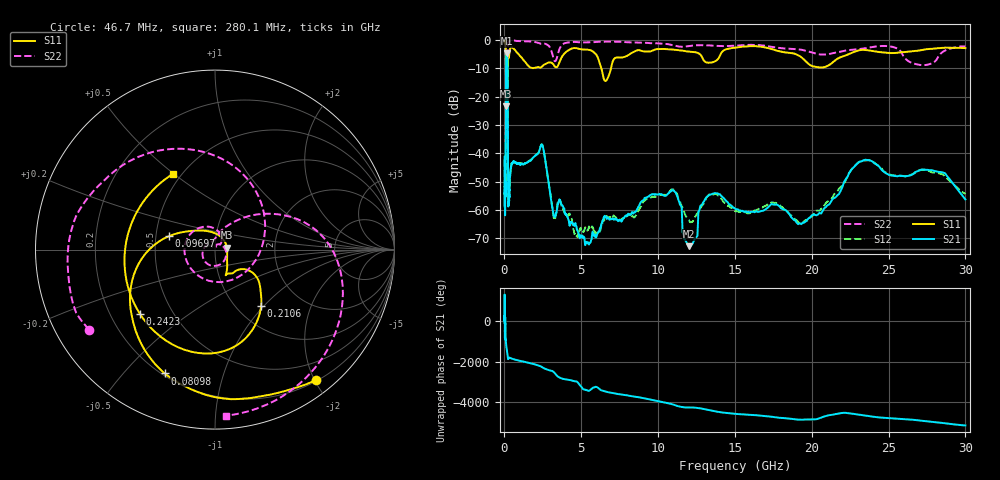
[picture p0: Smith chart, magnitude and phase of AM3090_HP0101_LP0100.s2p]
! Date/Time: Thu, Feb 28, 2019 1:58 PM
! Network Analyzer: Agilent Technologies E8364B Rev: A.07.50.67
! Sweep from 0.010 to 30.000 GHz, 1601 Points, Sweep Type: LOG
! Power Supply: 5.023 V, 0.002 A
# Hz S DB R 50
!freq MagS11 AngS11 MagS21 AngS21 MagS12 AngS12 MagS22 AngS22
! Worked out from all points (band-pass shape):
!   1601 points, 10 MHz to 30 GHz, reference 50 ohm
!   highest |S21| = -4.62 dB at 146.9 MHz (marker M1); lowest = -72.8 dB at 12.01 GHz (marker M2)
!   |S21| within 3 dB of the highest: 106.9 MHz to 197.1 MHz (90.2 MHz wide, 59.3 % of centre)
!   lowest |S11| = -23.4 dB at 105.1 MHz (marker M3), VSWR 1.14, Z = 57.1 + j1.3 ohm
!   |S11| at or under -10 dB: 96.08 MHz to 200.4 MHz (104.3 MHz wide, 70.4 % of centre); 6.307 GHz to 6.931 GHz (624.1 MHz wide, 9.43 % of centre)
!   |S22| runs from -34.9 to -0.1 dB; largest |S21 - S12| = 0.012
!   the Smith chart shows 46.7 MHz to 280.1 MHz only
!   S11 on the Smith chart (normalised r, x): 46.7 MHz: 0.22, -2.02; 80.98 MHz: 0.21, -0.65; 96.97 MHz: 0.58, +0.09; 210.6 MHz: 1.28, -0.96; 242.3 MHz: 0.33, -0.33; 280.1 MHz: 0.45, +0.49
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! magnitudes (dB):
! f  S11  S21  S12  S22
! 10 MHz  -0.3  -41.2  -42.2  -0.6
! 38.04 MHz  -0.5  -59.4  -60.7  -1.3
! 46.7 MHz  -0.8  -51.0  -50.0  -1.6
! 80.98 MHz  -2.6  -49.3  -49.0  -5.2
! 96.97 MHz  -11.4  -15.9  -15.9  -15.0
! 105.1 MHz  -23.4  -8.3  -8.3  -15.9
! 130.3 MHz  -16.3  -4.9  -4.9  -34.8
! 144.7 MHz  -16.3  -4.6  -4.6  -25.6
! 146.9 MHz  -16.2  -4.6  -4.6  -24.5
! 210.6 MHz  -7.8  -14.0  -13.9  -11.0
! 242.3 MHz  -5.2  -56.8  -54.5  -1.5
! 280.1 MHz  -6.3  -57.1  -57.4  -0.6
! 550.5 MHz  -2.9  -43.1  -43.1  -0.2
! 2.084 GHz  -9.7  -40.5  -40.4  -0.8
! 5.392 GHz  -3.4  -71.7  -67.3  -0.8
! 7.926 GHz  -5.7  -62.2  -62.4  -0.8
! 10.86 GHz  -3.3  -53.2  -52.7  -1.7
! 12.01 GHz  -4.1  -72.8  -63.5  -2.2
! 13.61 GHz  -7.8  -54.2  -54.6  -2.0
! 19.61 GHz  -7.5  -64.1  -63.5  -3.8
! 23.48 GHz  -3.5  -42.3  -42.6  -2.9
! 30 GHz  -2.9  -56.3  -54.3  -2.2
